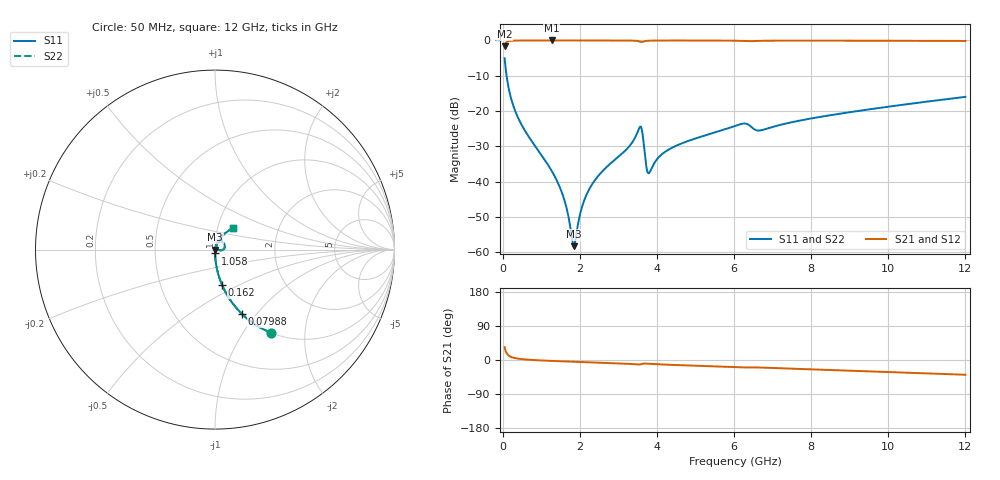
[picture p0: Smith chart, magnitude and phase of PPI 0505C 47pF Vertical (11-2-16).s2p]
# GHz S MA R 50
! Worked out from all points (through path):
!   1601 points, 50 MHz to 12 GHz, reference 50 ohm
!   highest |S21| = -0.01 dB at 1.275 GHz (marker M1); lowest = -1.6 dB at 50 MHz (marker M2)
!   group delay of S21, straight-line fit = 9.73 ps
!   lowest |S11| = -58.2 dB at 1.843 GHz (marker M3), VSWR 1.00, Z = 50.1 - j0.0167 ohm
!   |S11| at or under -10 dB: 101 MHz to end of sweep
!   |S22| runs from -58.2 to -5.0 dB; largest |S21 - S12| = 0
!   S11 on the Smith chart (normalised r, x): 50 MHz: 1.00, -1.35; 79.88 MHz: 1.00, -0.84; 162 MHz: 1.00, -0.41; 1.058 GHz: 1.00, -0.04; 12 GHz: 1.19, +0.30
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0.05  0.5594 -56.1  0.8287 33.9  0.8287 33.9  0.5594 -56.1
0.079875  0.3888 -67.3  0.921 22.7  0.921 22.7  0.3888 -67.3
0.1620312  0.2025 -78.6  0.9788 11.3  0.9788 11.3  0.2025 -78.6
0.4458437  0.07126 -86.5  0.9968 2.9  0.9968 2.9  0.07126 -86.5
1.058281  0.02169 -89.0  0.9988 -1.5  0.9988 -1.5  0.02169 -89.0
1.274875  0.01413 -88.3  0.9988 -2.4  0.9988 -2.4  0.01413 -88.3
1.588563  0.005785 -82.4  0.9987 -3.7  0.9987 -3.7  0.005785 -82.4
1.8425  0.001226 -7.8  0.9987 -4.7  0.9987 -4.7  0.001226 -7.8
2.044156  0.004157 66.4  0.9986 -5.4  0.9986 -5.4  0.004157 66.4
2.387719  0.01045 75.4  0.9984 -6.7  0.9984 -6.7  0.01045 75.4
3.269031  0.03109 73.3  0.9957 -10.1  0.9957 -10.1  0.03109 73.3
3.545375  0.05807 44.5  0.9664 -11.8  0.9664 -11.8  0.05807 44.5
3.612594  0.05345 9.9  0.9494 -10.2  0.9494 -10.2  0.05345 9.9
3.724625  0.01657 2.6  0.9836 -9.7  0.9836 -9.7  0.01657 2.6
3.776906  0.01317 29.1  0.9895 -10.1  0.9895 -10.1  0.01317 29.1
4.038312  0.02197 69.2  0.996 -11.5  0.996 -11.5  0.02197 69.2
4.598469  0.03409 72.3  0.9967 -13.6  0.9967 -13.6  0.03409 72.3
6.025  0.06153 64.9  0.9909 -18.8  0.9909 -18.8  0.06153 64.9
6.674781  0.05321 57.2  0.9862 -19.8  0.9862 -19.8  0.05321 57.2
8.019156  0.07895 62.9  0.9931 -24.7  0.9931 -24.7  0.07895 62.9
10.01331  0.1156 56.7  0.9894 -31.7  0.9894 -31.7  0.1156 56.7
12  0.1589 49.7  0.9829 -39.0  0.9829 -39.0  0.1589 49.7
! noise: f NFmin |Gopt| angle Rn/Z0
0.05  0.0003782  0.8611  0.5621  0.0005833
1.372  0.003863  0.6654  3.555  0.002211
2.701  0.00676  0.6315  6.781  0.003434
4.031  0.01216  0.6848  10.15  0.007428
5.36  0.01241  0.6088  13.24  0.005803
6.682  0.02808  0.7641  16.77  0.02367
8.012  0.01672  0.5768  19.47  0.006981
9.341  0.01778  0.5465  22.32  0.006742
10.67  0.01962  0.5357  25.16  0.007149
12  0.02172  0.5318  27.95  0.00775
